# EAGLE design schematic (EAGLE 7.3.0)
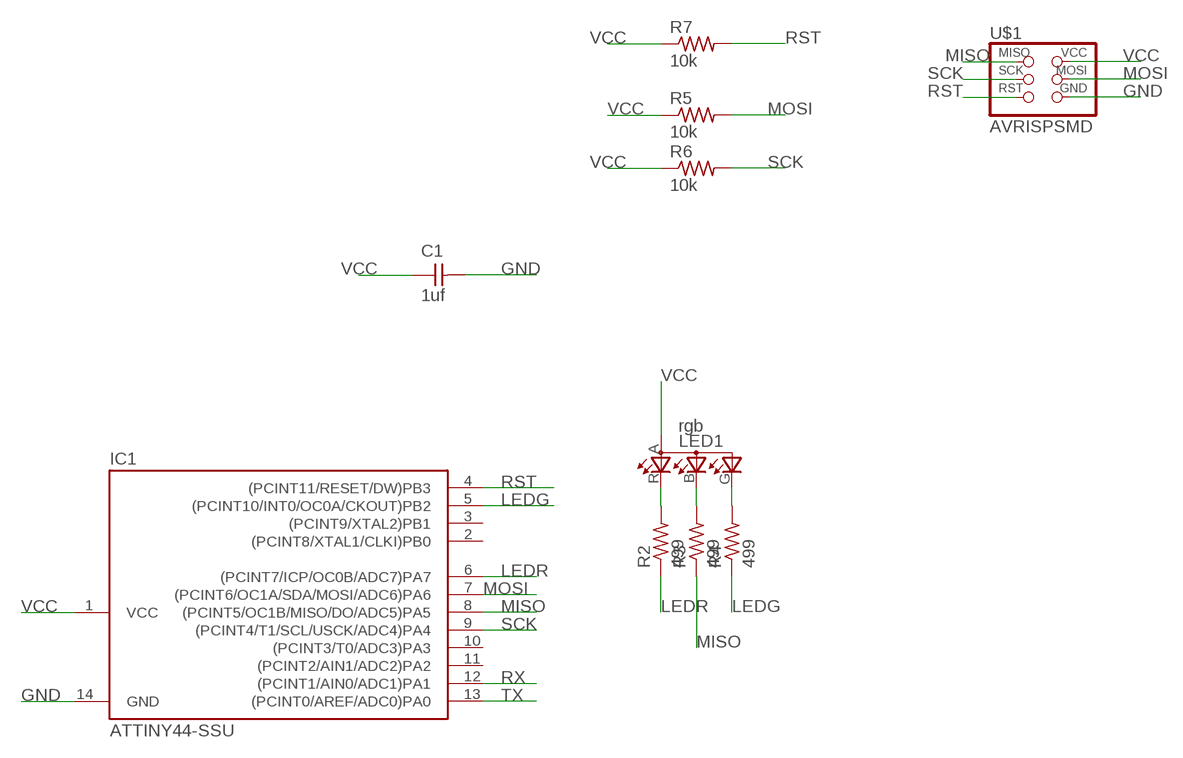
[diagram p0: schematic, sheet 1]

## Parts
C1  1uf  CAP-UNPOLARIZEDFAB  [C1206FAB]
IC1  ATTINY44-SSU  [SOIC14]
LED1  rgb  LEDRGBOLD  [P-LCC-4-3]
R2  499  RES-US1206FAB  [R1206FAB]
R3  499  RES-US1206FAB  [R1206FAB]
R4  499  RES-US1206FAB  [R1206FAB]
R5  10k  RES-US1206FAB  [R1206FAB]
R6  10k  RES-US1206FAB  [R1206FAB]
R7  10k  RES-US1206FAB  [R1206FAB]
U$1  AVRISPSMD  [2X03SMD]

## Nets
GND: C1.2 IC1.14(GND) U$1.6(GND)
LEDG: IC1.5((PCINT10/INT0/OC0A/CKOUT)PB2) R4.1
LEDR: IC1.6((PCINT7/ICP/OC0B/ADC7)PA7) R2.1
MISO: IC1.8((PCINT5/OC1B/MISO/DO/ADC5)PA5) R3.1 U$1.1(MISO)
MOSI: IC1.7((PCINT6/OC1A/SDA/MOSI/ADC6)PA6) R5.2 U$1.4(MOSI)
N$2: LED1.R(CRED) R2.2
N$3: LED1.B(CBLUE) R3.2
N$4: LED1.G(CGREEN) R4.2
RST: IC1.4((PCINT11/RESET/DW)PB3) R7.2 U$1.5(RST)
RX: IC1.12((PCINT1/AIN0/ADC1)PA1)
SCK: IC1.9((PCINT4/T1/SCL/USCK/ADC4)PA4) R6.2 U$1.3(SCK)
TX: IC1.13((PCINT0/AREF/ADC0)PA0)
VCC: C1.1 IC1.1(VCC) LED1.A(A2) R5.1 R6.1 R7.1 U$1.2(VCC)
Unconnected: IC1.2((PCINT8/XTAL1/CLKI)PB0) IC1.3((PCINT9/XTAL2)PB1) IC1.10((PCINT3/T0/ADC3)PA3) IC1.11((PCINT2/AIN1/ADC2)PA2)

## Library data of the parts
C1 = 02fab:CAP-UNPOLARIZED
IC1 = 01_fab:ATTINY44
LED1 = 02fab:LEDRGBOLD: OSRAM Hyper Multi TOPLED® Hyper-Bright LED LATB T686 Source: http://www.osram.convergy.de/
R2-R7 = 02fab:RES-US: Resistor (US Symbol)
U$1 = 02fab:AVRISP

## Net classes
0 default: width 0.4 mm, drill 0.4 mm, clearance 0.406 mm

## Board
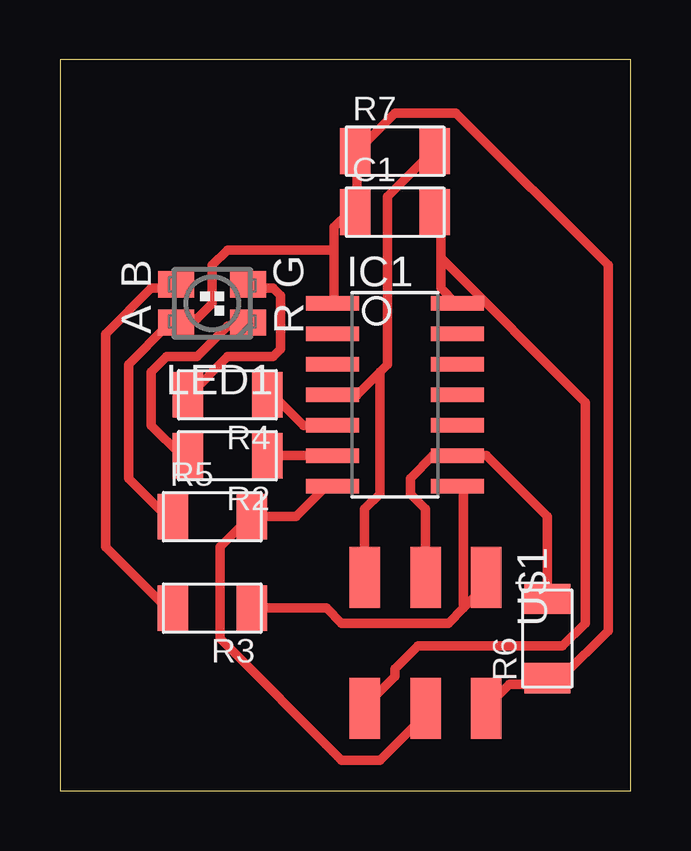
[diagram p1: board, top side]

Size 23.8 x 30.47 mm. Coordinates in mm from the lower left corner, seen from the top.
Outline: 0,0 23.8,0 23.8,30.47 0,30.47 0,0
Copper layers (1*16): Top 0.035mm / dielectric 1.5mm / Bottom 0.035mm
Design rules "default *": minimum track width 10mil, minimum drill 24mil, track to track 16mil, track to pad 16mil, pad to pad 16mil, via to via 16mil, smd to smd 16mil, copper to edge 40mil, drill to drill 8mil, minimum pad ring 10mil, minimum via ring 8mil, stop-mask expansion 4mil, vias tented up to drill 0mil, thermal gap 10mil

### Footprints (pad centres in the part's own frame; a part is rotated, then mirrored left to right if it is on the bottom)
C1206FAB = smd 1.27 x 1.905: 1 -1.651,0; 2 1.651,0
SOIC14 = smd 0.61 x 2.21: 1 -3.81,-2.603; 2 -2.54,-2.603; 3 -1.27,-2.603; 4 0,-2.603; 5 1.27,-2.603; 6 2.54,-2.603; 7 3.81,-2.603; 8 3.81,2.603; 9 2.54,2.603; 10 1.27,2.603; 11 0,2.603; 12 -1.27,2.603; 13 -2.54,2.603; 14 -3.81,2.603
P-LCC-4-3 = smd 1.1 x 1.5: A -0.8,1.5; B 0.8,1.5; G 0.8,-1.5; R -0.8,-1.5
R1206FAB = smd 1.27 x 1.905: 1 -1.651,0; 2 1.651,0
2X03SMD = smd 2.54 x 1.27: 1 -2.54,2.54; 2 2.92,2.54; 3 -2.54,0; 4 2.92,0; 5 -2.54,-2.54; 6 2.92,-2.54

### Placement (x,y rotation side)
C1  13.97,24.13 0 top
IC1  13.97,16.51 270 top
LED1  6.35,20.32 90 top
R2  6.99,13.97 180 top
R3  6.35,7.62 180 top
R4  6.99,16.51 180 top
R5  6.35,11.43 0 top
R6  20.32,6.35 90 top
R7  13.97,26.67 0 top
U$1  15.24,6.35 270 top

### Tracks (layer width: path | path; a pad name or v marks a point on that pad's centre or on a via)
GND
  Top 0.4: 15.88,22.23 15.88,20.96 16.51,20.32 IC1.14 | 15.88,22.23 15.88,24.13 C1.2 | 15.88,22.23 21.91,16.19 21.91,6.99 20.96,6.03 14.92,6.03 13.97,5.08 13.97,4.76 12.7,3.49 U$1.6
LEDG
  Top 0.4: IC1.5 10.16,15.24 8.89,16.51 R4.1
LEDR
  Top 0.4: IC1.6 R2.1
MISO
  Top 0.4: R3.1 11.11,7.62 11.75,6.99 16.19,6.99 16.83,7.62 | 16.83,7.62 17.78,8.57 U$1.1 | 16.83,7.62 16.83,12.7 IC1.8
MOSI
  Top 0.4: IC1.7 11.11,12.7 9.84,11.43 R5.2 7.94,11.43 6.67,10.16 6.67,6.35 11.75,1.27 13.34,1.27 15.24,3.18 U$1.4
N$2
  Top 0.4: LED1.R 7.62,19.37 6.99,19.37 5.71,18.1 4.45,18.1 3.81,17.46 3.81,15.24 5.08,13.97 R2.2
N$3
  Top 0.4: LED1.B 4.76,20.96 3.81,20.96 1.9,19.05 1.9,10.16 4.45,7.62 R3.2
N$4
  Top 0.4: LED1.G 7.94,20.96 8.89,20.96 9.21,20.64 9.21,18.41 8.89,18.1 6.99,18.1 5.4,16.51 R4.2
RST
  Top 0.4: 13.34,17.46 12.38,16.51 IC1.4 | 13.34,17.46 13.65,17.78 13.65,24.77 15.56,26.67 R7.2 | U$1.5 12.7,11.75 13.34,12.38 13.34,17.46
SCK
  Top 0.4: R6.2 20.32,11.43 17.78,13.97 IC1.9 15.56,13.97 14.61,13.02 14.61,12.38 15.24,11.75 U$1.3
VCC
  Top 0.4: R5.1 4.45,11.43 2.86,13.02 2.86,17.78 4.45,19.37 4.76,19.37 LED1.A 5.08,19.68 5.71,19.68 6.35,20.32 6.35,21.91 6.99,22.54 11.43,22.54 | U$1.2 17.78,3.49 18.73,4.45 20.32,4.45 R6.1 20.32,4.76 20.96,4.76 22.86,6.67 22.86,21.91 16.51,28.26 13.97,28.26 12.38,26.67 | 12.38,26.67 12.38,24.13 C1.1 12.07,24.13 11.43,23.5 11.43,22.54 | 11.43,22.54 11.43,20.32 IC1.1 | 12.38,26.67 R7.1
